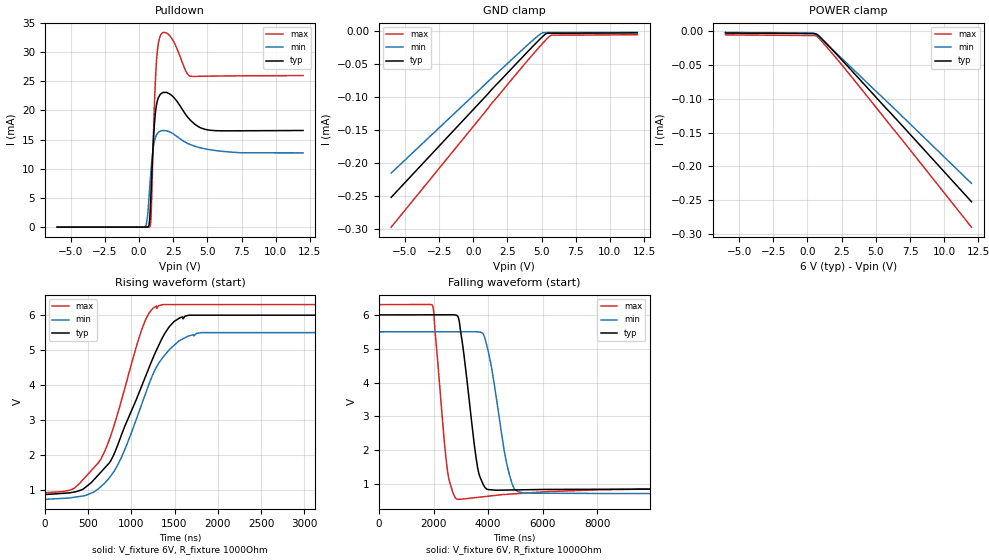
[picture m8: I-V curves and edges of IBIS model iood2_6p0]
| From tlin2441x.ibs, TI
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|   iood2_6p0 Model
[Model]   iood2_6p0
Model_type   I/O_open_drain
Polarity   Non-Inverting
Enable   Active-Low
Vinl = 1.2
Vinh = 5.1
Vmeas = 3
Vref = 6
Cref = 2pF
Rref = 1000
|   typ   min   max
C_comp   7.685pF   7.510pF   8.465pF
|  Where Nom  PVT is Nominal Process, 6.0V,   27C
|   Fast PVT is Strong Process,  6.3V,   -40C
|   Slow PVT is Weak Process,   5.5V,   150C
[Model spec]
|subparameter
Vinl   1.2   1.1   1.26
Vinh   5.1   4.675   5.355
[Voltage Range]   6   5.5   6.3
|Junction Temperature
[Temperature Range]   27   150   -40
[Pullup Reference]   6   5.5   6.3
[Pulldown Reference]   -0   0   -0
[Power Clamp Reference]   6   5.5   6.3
[GND Clamp Reference]   0   0   0
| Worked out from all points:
|   slope of the pulldown table from 0 to 0.9 V, typ, clamps not added: 120 ohm
|   falling waveform, V_fixture 6V, R_fixture 1000Ohm: 20-80 % time 450ns typ, 561ns min, 340ns max; typ from 6 V to 0.857 V
|   rising waveform, V_fixture 6V, R_fixture 1000Ohm: 20-80 % time 511ns typ, 463ns min, 402ns max; typ from 0.857 V to 6 V
[Pulldown]
|   Voltage   I(typ)   I(min)   I(max)
-6V       -813.1nA   -1.156uA   -712.9nA
354mV     -257.4nA   6.263uA    -242.1nA
624mV     12.58uA    1.953mA    -114.8nA
786mV     1.727mA    7.102mA    61.57uA
894mV     7.164mA    10.39mA    2.888mA
1.11V     17.29mA    14.56mA    20.16mA
1.254V    20.65mA    15.71mA    27.74mA
1.416V    22.19mA    16.24mA    31.56mA
1.704V    23.01mA    16.54mA    33.28mA
2.424V    22.48mA    16.09mA    32.2mA
3.684V    18.49mA    14.21mA    25.91mA
12V       16.56mA    12.72mA    25.96mA
[GND Clamp]
|   Voltage   I(typ)   I(min)   I(max)
-6V       -252.1uA   -215.2uA   -297.3uA
1.308V    -89.38uA   -71.84uA   -110.5uA
4.296V    -24.22uA   -14.81uA   -36.67uA
5.052V    -8.471uA   -2.572uA   -18.93uA
5.34V     -3.677uA   -1.968uA   -12.52uA
5.61V     -2.949uA   -1.962uA   -7.247uA
5.808V    -2.943uA   -1.957uA   -5.886uA
12V       -2.481uA   -1.599uA   -5.232uA
[POWER Clamp]
|   Voltage   I(typ)   I(min)   I(max)
-6V       -2.763uA   -1.916uA   -5.468uA
264mV     -3.703uA   -2.82uA    -6.61uA
462mV     -3.73uA    -3.51uA    -6.639uA
696mV     -4.891uA   -6.669uA   -8.088uA
1.344V    -17.41uA   -18.23uA   -21.94uA
3.036V    -54.09uA   -50.53uA   -62.86uA
12V       -252.1uA   -225uA     -289.7uA
[Ramp]
R_load = 1000
|   typ   min   max
dV/dt_r   3.08746/5.10931e-07   2.86908/4.62693e-07   3.23848/4.02243e-07
dV/dt_f   3.08746/4.49246e-07   2.86908/5.60576e-07   3.23848/3.38908e-07
[Falling Waveform]
V_fixture = 6V
V_fixture_min = 5.5V
V_fixture_max = 6.3V
R_fixture = 1000Ohm
C_fixture = 0F
|   Time   V(typ)   V(min)   V(max)
0s        6.003V     5.502V     6.306V
1.967us   6.005V     5.504V     6.275V
2.504us   6.006V     5.504V     1.427V
2.862us   5.98V      5.504V     554.8mV
3.091us   4.958V     5.505V     561.6mV
3.616us   1.472V     5.501V     609mV
4.006us   838.8mV    4.914V     644.1mV
4.75us    826mV      1.362V     702.1mV
5.293us   833mV      736mV      731.7mV
50us      857.5mV    720.5mV    908.6mV
[Rising Waveform]
V_fixture = 6V
V_fixture_min = 5.5V
V_fixture_max = 6.3V
R_fixture = 1000Ohm
C_fixture = 0F
|   Time   V(typ)   V(min)   V(max)
0s        857.5mV    720.5mV    908.6mV
347.6ns   933.5mV    782.8mV    1.053V
619.2ns   1.421V     1.022V     1.769V
744.3ns   1.759V     1.327V     2.42V
893.2ns   2.609V     1.961V     3.619V
1.154us   4.177V     3.677V     5.804V
1.368us   5.393V     4.798V     6.303V
1.564us   5.927V     5.278V     6.303V
1.813us   5.999V     5.5V       6.303V
50us      6.003V     5.502V     6.306V
